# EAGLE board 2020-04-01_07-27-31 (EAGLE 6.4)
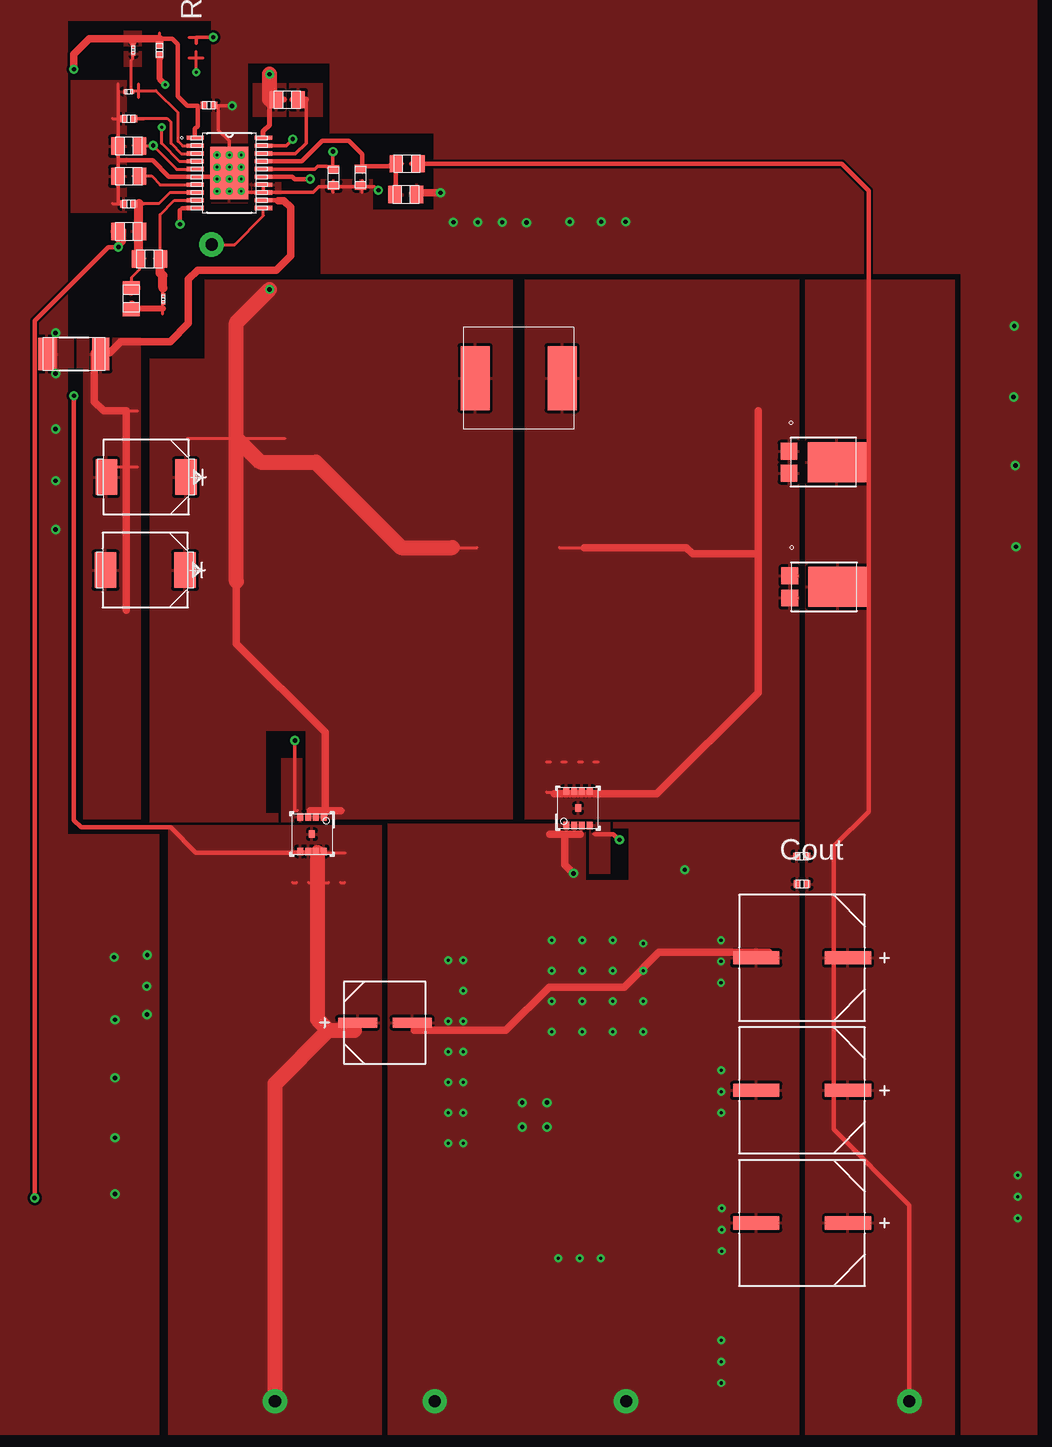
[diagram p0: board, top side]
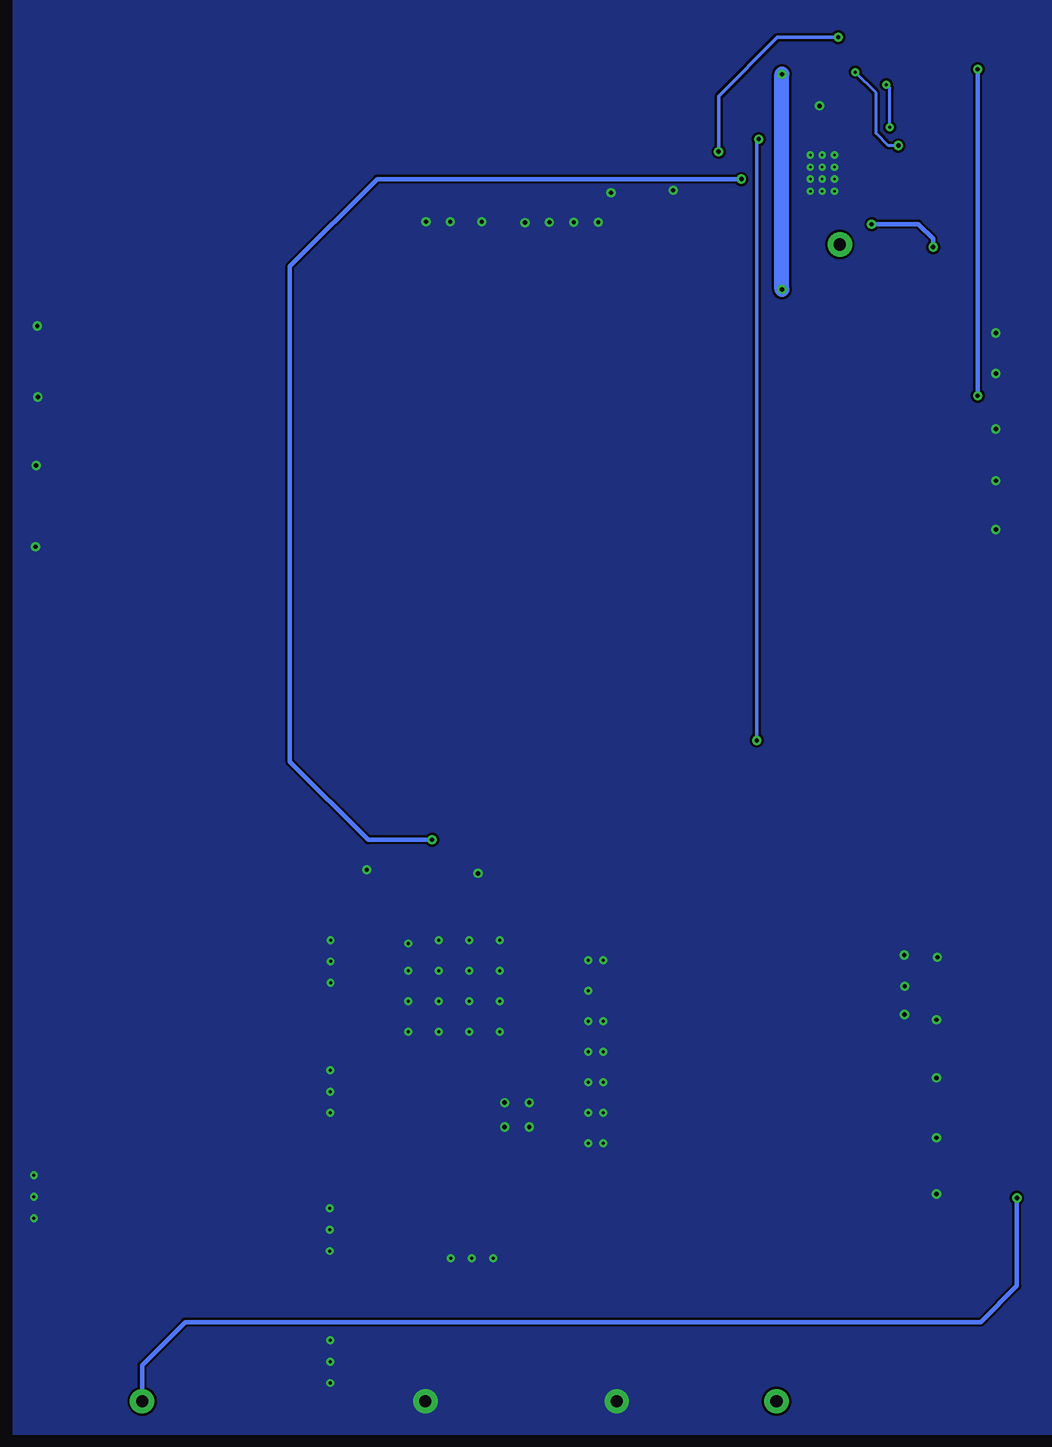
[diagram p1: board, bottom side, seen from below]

No outline drawn. Coordinates in mm, seen from the top.
Copper layers ((1*2)+(15*16)): TOP / INTERNAL1 / layer 15 / BOTTOM

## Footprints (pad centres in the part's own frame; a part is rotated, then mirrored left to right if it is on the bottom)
0805 = smd 1.118 x 1.448: 1 -0.902,0; 2 0.902,0
CAPSMT_62_C10 = smd 3.251 x 0.813: 1 -2.273,0; 2 2.273,0
0402 = smd 0.559 x 0.61: 1 -0.419,0; 2 0.419,0
CAPSMT_62_F12 = smd 3.861 x 1.092: 1 -3.823,0; 2 3.823,0
0603 = smd 0.66 x 0.965: 1 -0.699,0; 2 0.699,0
SMC = smd 1.803 x 2.972: 1 -3.315,0; 2 3.315,0
PowerDI5 = smd 1.397 x 1.397: 1 -0.92,-2.857; 3 0.92,-2.857 | smd 3.353 x 4.851: 2 0,1.13
TP-1502 = drill 0.813 round: 1 0,0
WE-LHMI_8040 = smd 2.42 x 5.33: 1 -3.62,0; 2 3.62,0
DQG0008A = smd 0.63 x 0.5: 1 -1.435,0.975; 2 -1.435,0.325; 3 -1.435,-0.325; 4 -1.435,-0.975; 5 1.435,-0.975; 6 1.435,-0.325; 7 1.435,0.325; 8 1.435,0.975; 9 0,0
0201 = smd 0.356 x 0.33: 1 -0.292,0; 2 0.292,0
2512 = smd 1.422 x 2.718: 1 -2.248,0; 2 2.248,0
MXA20A = smd 1.422 x 0.356: 1 -2.845,2.925; 2 -2.845,2.275; 3 -2.845,1.625; 4 -2.845,0.975; 5 -2.845,0.325; 6 -2.845,-0.325; 7 -2.845,-0.975; 8 -2.845,-1.625; 9 -2.845,-2.275; 10 -2.845,-2.925; 11 2.845,-2.925; 12 2.845,-2.275; 13 2.845,-1.625; 14 2.845,-0.975; 15 2.845,-0.325; 16 2.845,0.325; 17 2.845,0.975; 18 2.845,1.625; 19 2.845,2.275; 20 2.845,2.925 | smd 3.15 x 4.343: 21 0,0

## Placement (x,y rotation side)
Cboot  [0805]  51.31,137.41 0 top
Ccomp  [0805]  39.83,124.16 180 top
Ccomp2  [0805]  38.3,120.85 90 top
Cin  [CAPSMT_62_C10]  59.44,60.5 0 top
Cinx  [0402]  44.78,136.96 0 top
Cout_1  [CAPSMT_62_F12]  94.21,65.91 180 top
Cout_2  [CAPSMT_62_F12]  94.21,54.86 180 top
Cout_3  [CAPSMT_62_F12]  94.21,43.81 180 top
Coutx  [0402]  94.21,72.06 180 top
Coutx2  [0402]  94.18,74.37 180 top
Cramp  [0805]  38.1,133.55 180 top
Css  [0805]  38.1,131.04 180 top
Cvcc  [0603]  55.17,130.94 270 top
Cvccx  [0603]  57.43,130.96 90 top
D1  [SMC]  39.47,98.22 180 top
D2  [PowerDI5]  96.04,96.82 270 top
D3  [SMC]  39.55,105.97 180 top
D4  [PowerDI5]  95.99,107.21 270 top
GND  [TP-1502]  63.58,28.91 180 top
GND1  [TP-1502]  79.53,28.91 180 top
L1  [WE-LHMI_8040]  70.59,114.22 180 top
M1  [DQG0008A]  53.37,76.23 270 top
M2  [DQG0008A]  75.54,78.38 90 top
Rcomp  [0201]  40.97,120.8 270 top
Renable  [0402]  40.67,141.55 270 top
Rfbb  [0402]  38.1,128.73 180 top
Rfbt  [0805]  38.1,126.44 0 top
RHIGH  [0805]  61.29,132.08 0 top
RLOW  [0805]  61.19,129.51 180 top
Rsense  [2512]  33.53,116.23 180 top
Rt  [0402]  38.1,135.84 180 top
Ruv1  [0201]  38.48,141.55 270 top
Ruv2  [0201]  38.1,138.1 180 top
Sync  [TP-1502]  44.96,125.35 180 top
U1  [MXA20A]  46.48,131.32 0 top
VIN  [TP-1502]  50.24,28.91 180 top
VOUT  [TP-1502]  103.12,28.91 180 top

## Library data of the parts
Cboot = ultra-librarian; RefDes: Cboot; Type: 08053C104JAZ2A
Ccomp = ultra-librarian; RefDes: Ccomp; Type: CL21C222JBFNNNE
Ccomp2 = ultra-librarian; RefDes: Ccomp2; Type: 08053C104JAZ2A
Cin = ultra-librarian; RefDes: Cin; Type: 16SVPG270M
Cinx = ultra-librarian; RefDes: Cinx; Type: GRM155R71C104KA88D
Cout_1-Cout_3 Coutx Coutx2 = ultra-librarian
Cramp = ultra-librarian; RefDes: Cramp; Type: CL21C471KBANNNC
Css = ultra-librarian; RefDes: Css; Type: CGA4J2C0G1H223J125AA
Cvcc = ultra-librarian; RefDes: Cvcc; Type: C0603C105Z8VACTU
Cvccx = ultra-librarian; RefDes: Cvccx; Type: C0603C105Z8VACTU
D1 = ultra-librarian; RefDes: D1; Type: B540C-13-F
D2 = ultra-librarian; RefDes: D2; Type: PDS760-13
D3 = ultra-librarian; RefDes: D3; Type: B540C-13-F
D4 = ultra-librarian; RefDes: D4; Type: PDS760-13
GND = ultra-librarian; RefDes: GND; Type: TP-1502
GND1 = ultra-librarian; RefDes: GND1; Type: TP-1502
L1 = ultra-librarian; RefDes: L1; Type: 74437358082
M1 = ultra-librarian; RefDes: M1; Type: CSD16340Q3
M2 = ultra-librarian; RefDes: M2; Type: CSD16340Q3
Rcomp = ultra-librarian; RefDes: Rcomp; Type: RC0201FR-0712K1L
Renable = ultra-librarian; RefDes: Renable; Type: CRCW04021M00FKED
Rfbb = ultra-librarian; RefDes: Rfbb; Type: CRCW04021K00FKED
Rfbt = ultra-librarian; RefDes: Rfbt; Type: RT0805BRD073K05L
RHIGH = ultra-librarian; RefDes: RHIGH; Type: 08051A100CAT2A
RLOW = ultra-librarian; RefDes: RLOW; Type: 08051A100CAT2A
Rsense = ultra-librarian; RefDes: Rsense; Type: PMR100HZPFU10L0
Rt = ultra-librarian; RefDes: Rt; Type: CRCW040261K9FKED
Ruv1 = ultra-librarian; RefDes: Ruv1; Type: RC0201FR-0712K1L
Ruv2 = ultra-librarian; RefDes: Ruv2; Type: RC0201FR-0712K1L
Sync = ultra-librarian; RefDes: Sync; Type: TP-1502
U1 = ultra-librarian; RefDes: U1; Type: LM25118MH/NOPB
VIN = ultra-librarian; RefDes: VIN; Type: TP-1502
VOUT = ultra-librarian; RefDes: VOUT; Type: TP-1502

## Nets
0: Cin.2 Cinx.2 Cout_1.2 Cout_2.2 Cout_3.2 Coutx2.2 Coutx.2 Cramp.2 Css.2 Cvcc.2 Cvccx.1 GND1.1 GND.1 M2.1 M2.2 M2.3 Rfbb.2 RLOW.1 Rsense.2 Rt.2 Ruv2.2 U1.6 U1.13 U1.14 U1.21
1: Ruv1.2 Ruv2.1 U1.2
2: Rt.1 U1.3
3: Renable.2 U1.4
4: Cramp.1 U1.5
5: Css.1 U1.7
6: Cout_1.1 Cout_2.1 Cout_3.1 Coutx2.1 Coutx.1 Cvccx.2 D2.2 D4.2 Rfbt.1 RHIGH.1 RHIGH.2 RLOW.2 U1.10 U1.17 VOUT.1
7: Ccomp2.2 Ccomp.2 Rfbb.1 Rfbt.2 U1.8
8: Ccomp.1 Rcomp.1 U1.9
9: Cin.1 Cinx.1 M1.5 M1.6 M1.7 M1.8 M1.9 Renable.1 Ruv1.1 U1.1 VIN.1
10: Cboot.1 D1.1 D3.1 L1.2 M1.1 M1.2 M1.3 U1.20
11: D1.2 D3.2 Rsense.1 U1.12
12: M2.4 U1.15
13: Ccomp2.1 Rcomp.2
14: Cvcc.1 U1.16
15: M1.4 U1.19
16: Cboot.2 U1.18
17: D2.1 D2.3 D4.1 D4.3 L1.1 M2.5 M2.6 M2.7 M2.8 M2.9
19: Sync.1 U1.11

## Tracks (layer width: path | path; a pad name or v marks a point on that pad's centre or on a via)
0  (via drill 0.2 pad 0.48, 0.25 pad 0.61, 0.36 pad 0.71, 1.02 pad 2.03)
  TOP 0.254: 55.1,129.69 55.1,130.63 | 57.54,129.69 57.54,130.63 | 37.22,137.59 37.22,138.74 | 36.75,131.05 37.69,131.05 | 36.75,133.59 37.69,133.59 | 75.56,76.24 75.84,76.24 | 74.3,76.24 74.57,76.24 | 73.03,76.24 73.3,76.24 | 36.75,128.76 37.69,128.76 | 46.46,129.39 46.46,133.22 | 36.75,135.85 37.69,135.85
  TOP 0.305: 37.69,128.78 37.24,128.78 37.24,130.94 | 37.24,131.06 37.24,133.6 37.24,135.87 | 45.29,130.99 v45.47,130.81 | U1.13 49.33,130.33 | U1.13 47.6,129.69 v47.47,129.79 | v46.48,132.82 46.48,133.99 45.57,134.87 45.57,136.91 v46.71,136.91 | 57.56,130.18 55.12,130.18 53.95,130.18 53.47,129.69 U1.13 | 37.24,135.87 | 37.24,135.87 37.24,138.18 | v58.9,129.87 58.57,130.18 57.56,130.18 | 32,116.33 v32,117.98 | 32,116.33 | v32,114.61 32,116.33 | 57.56,130.18 57.56,130.66
  TOP 0.356: 37.39,132.36 40.08,132.36 41.43,130.99 43.61,130.99 45.29,130.99
  TOP 0.635: 91.44,66.37 82.27,66.37 79.38,63.48 73.13,63.48 69.52,59.87 61.9,59.87 | v64.08,129.67 62.08,129.67 61.77,129.67 | 73.18,76.22 74.45,76.22 | 74.45,76.22 75.72,76.22 | 74.45,76.22 74.45,73.66 v75.16,72.95
  other vias: 46.48,131.8 47.47,131.8 46.48,130.81 47.47,130.81 46.48,129.79 45.47,129.79 45.47,131.8 45.47,132.82 47.47,132.82 111.89,118.57 111.84,112.65 65.99,65.71 65.99,63.17 65.99,60.63 65.99,58.09 64.72,50.47 65.99,55.55 65.99,53.01 65.99,50.47 64.72,65.71 64.72,60.63 64.72,58.09 64.72,55.55 64.72,53.01 39.65,66.14 36.96,60.76 36.96,50.93 36.96,55.91 36.88,65.96 77.47,127.25 79.5,127.25 112.04,100.18 111.99,106.93 39.62,61.19 39.6,63.55 32,101.6 32,105.66 32,109.98 74.85,127.25 36.96,46.23 70.89,53.85 70.89,51.82 72.95,53.85 72.95,51.82 84.43,73.25 71.25,127.18 67.18,127.2 65.15,127.2 69.22,127.2 87.45,63.83 87.45,67.39 87.45,65.61 87.48,52.98 87.48,56.54 87.48,54.76 87.48,30.48 87.48,34.04 87.48,32.26 87.5,41.48 87.5,45.03 87.5,43.26 73.36,59.74 73.36,62.28 73.36,64.82 75.9,59.74 75.9,62.28 75.9,64.82 78.44,64.82 78.44,62.28 78.44,59.74 80.98,59.74 80.98,62.28 80.98,64.82 78.44,67.36 75.9,67.36 73.36,67.36 80.98,67.11 112.17,46 112.17,47.78 112.17,44.22 73.89,40.87 77.44,40.87 75.67,40.87 63.6,28.96 79.55,28.96
  pour TOP (rank 6): 42.93,130.81 42.93,131.14 44.09,131.14 44.09,130.81
  pour TOP (rank 6): 48.62,129.51 48.62,129.84 49.81,129.84 49.81,129.51
  pour TOP (rank 6): 61.42,128.91 61.42,130.4 62.71,130.4 62.71,128.91
  pour TOP: 63.5,134.62 54.86,134.62 54.86,140.46 48.01,140.46 48.01,130.56 50.8,130.56 50.8,129.54 48.01,129.54 48.01,128.78 44.96,128.78 44.96,144.02 33.02,144.02 33.02,117.6 33.53,117.6 33.53,115.06 33.02,115.06 33.02,76.2 40.64,76.2 40.64,26.16 26.16,26.16 26.16,154.18 113.79,154.18 113.79,26.16 107.44,26.16 107.44,122.94 54.1,122.94 54.1,130.81 58.42,130.81 58.42,128.27 63.5,128.27
  pour TOP: 59.69,77.09 76.2,77.09 76.2,72.39 79.76,72.39 79.76,76.71 78.49,76.71 78.49,77.22 93.98,77.22 93.98,26.16 59.69,26.16
  pour TOP: 37.92,139.04 37.92,127.99 33.27,127.99 33.27,136.4 33.27,136.93 33.27,139.04
  pour BOTTOM: 113.92,154.43 113.92,26.16 25.91,26.16 25.91,154.43
1
  TOP 0.254: 38.43,141.35 38.43,140.82 38.3,140.69 38.3,138.33 38.46,138.18 38.94,138.18 40.36,138.18 42.22,136.32 42.22,133.96 42.6,133.58 43.61,133.58 | 38.92,137.59 38.92,138.74
  pour TOP: 42.93,133.4 42.93,133.73 44.09,133.73 44.09,133.4
  pour TOP (rank 5): 37.67,140.16 37.67,141.45 39.17,141.45 39.17,140.16
2
  TOP 0.254: 43.61,132.92 42.47,132.92 41.63,133.78 41.63,135.53 41.3,135.87 38.94,135.87 38.35,135.87 | 38.46,135.85 39.4,135.85
  pour TOP (rank 2): 42.93,132.77 42.93,133.1 44.09,133.1 44.09,132.77
3  (via drill 0.25 pad 0.61)
  TOP 0.254: v40.84,135.13 40.84,133.78 42.32,132.28 43.61,132.28 | 40.68,140.34 40.68,141.28
  TOP 0.508: 40.69,141.25 40.69,140.82 40.69,139.14 v41.15,138.68
  BOTTOM 0.254: v41.15,138.68 40.84,138.38 v40.84,135.13
  pour TOP (rank 2): 42.93,132.11 42.93,132.44 44.09,132.44 44.09,132.11
4  (via drill 0.25 pad 0.61, 0.36 pad 0.71)
  TOP 0.254: 43.61,131.62 42.09,131.62 v40.13,133.6 38.94,133.6 38.61,133.6 | v43.71,139.72 43.71,140.92 43.71,141.45 | 38.46,133.59 39.4,133.59 | 43.13,140.91 44.27,140.91
  BOTTOM 0.254: v43.71,139.72 41.99,138 41.99,134.62 40.97,133.6 v40.13,133.6
  pour TOP (rank 2): 42.93,131.44 42.93,131.78 44.09,131.78 44.09,131.44
5
  TOP 0.254: 43.61,130.33 40.72,130.33 40.01,131.06 38.94,131.06 38.56,131.06 | 38.46,131.05 39.4,131.05
  pour TOP (rank 2): 42.93,130.15 42.93,130.48 44.09,130.48 44.09,130.15
6  (via drill 0.36 pad 0.71, 1.02 pad 2.03)
  TOP 0.254: 57.54,131.39 57.54,132.33 | 61.57,132.07 62.51,132.07 | 59.87,132.07 60.81,132.07
  TOP 0.356: 37.69,126.59 37.69,125.58 v37.24,125.15 | v37.24,125.15 36.4,125.15 30.25,119 v30.25,45.9 | v37.24,125.15 37.24,126.47 | 60.38,129.16 60.38,129.67 60.35,129.69 60.35,132.08 | 60.35,132.08 60.17,131.88 57.56,131.88 | 99.75,97.28 99.75,78.11 96.85,75.21 96.85,51.61 103.15,45.31 v103.15,28.96 | 99.75,97.28 | 99.75,97.28 99.75,109.22 99.75,129.84 97.54,132.08 62.05,132.08 61.62,132.08 | 57.56,131.88 57.56,132.89 56.44,134.01 54.23,134.01 52.5,132.28 U1.17 | v42.37,127.05 42.37,128.19 42.55,128.37 43.61,128.37 | 57.56,131.42 57.56,131.88 | 60.35,132.08 60.83,132.08
  BOTTOM 0.356: v42.37,127.05 38.46,127.05 37.24,125.83 v37.24,125.15 | v30.25,45.9 30.25,38.58 33.27,35.56 99.57,35.56 103.15,31.98 v103.15,28.96
  pour TOP: 36.58,125.7 36.58,127.2 37.87,127.2 37.87,125.7
  pour TOP (rank 3): 42.93,128.19 42.93,128.52 44.09,128.52 44.09,128.19
  pour TOP (rank 3): 48.62,132.11 48.62,132.44 49.81,132.44 49.81,132.11
  pour TOP (rank 4): 59.72,128.91 59.72,130.4 61.01,130.4 61.01,128.91
  pour TOP (rank 5): 94.49,122.43 106.93,122.43 106.93,26.16 94.49,26.16
7
  TOP 0.254: 38.94,128.78 | 38.94,128.78 38.91,128.75 38.41,128.75 | 43.61,129.69 41.55,129.69 40.64,128.78 38.94,128.78 | 39.01,123.29 38.35,122.63 38.35,121.74 38.35,121.23 | 39.01,123.29 | 39.01,123.29 39.01,124.21 | 38.53,124.19 39.47,124.19 | 38.46,128.76 39.4,128.76
  TOP 0.762: 38.94,128.78 38.94,126.47 38.94,124.28 39.01,124.21
  pour TOP: 38.28,125.7 38.28,127.2 39.57,127.2 39.57,125.7
  pour TOP: 37.59,121.08 37.59,122.38 39.09,122.38 39.09,121.08
  pour TOP (rank 2): 42.93,129.51 42.93,129.84 44.09,129.84 44.09,129.51
8
  TOP 0.254: 43.61,129.03 41.91,129.03 40.72,127.84 40.72,124.21 | 40.93,121.26 40.93,122.2 | 40.23,124.19 41.17,124.19
  TOP 0.762: 40.95,121.74 40.95,122.76 40.72,122.99 40.72,124.21
  pour TOP (rank 2): 42.93,128.85 42.93,129.18 44.09,129.18 44.09,128.85
9  (via drill 0.36 pad 0.71, 1.02 pad 2.03)
  TOP 0.254: 55.75,72.17 56.08,72.17 | 54.43,72.17 54.76,72.17 | 53.09,72.17 53.42,72.17 | 51.77,72.17 52.09,72.17 | 51.77,74.66 56.11,74.66 | 40.68,142.04 40.68,142.98
  TOP 0.356: 40.69,142.52 41.71,142.52 42.19,142.04 42.19,137.69 42.98,136.91 43.87,136.91 43.87,135.23 43.61,135 43.61,134.24 | 53.85,74.68 43.69,74.68 41.6,76.78 34.14,76.78 33.53,77.39 v33.53,112.75
  TOP 0.635: v33.53,139.95 33.53,141.22 34.82,142.52 38.43,142.52 | 38.43,142.19 38.43,142.52 | 40.69,142.19 40.69,142.52 38.43,142.52 | 40.69,142.19
  TOP 1.27: 53.85,74.68 53.85,60.76 54.74,59.87 | 54.74,59.87 56.9,59.87 | 54.74,59.87 50.29,55.42 v50.29,28.96
  BOTTOM 0.356: v33.53,112.75 v33.53,139.95
  pour TOP: 42.93,134.06 42.93,134.39 44.09,134.39 44.09,134.06
  pour TOP (rank 5): 37.67,141.86 37.67,143.15 39.17,143.15 39.17,141.86
  pour TOP (rank 6): 59.18,26.16 59.18,76.96 41.4,76.96 41.4,26.16
10  (via drill 0.36 pad 0.71)
  TOP 0.254: 53.16,78.17 53.44,78.17 | 54.43,78.17 54.71,78.17 | 55.7,78.17 55.98,78.17 | 62.99,100.09 67.13,100.09 | 43,109.21 51.13,109.21
  TOP 0.406: 49.84,137.44 49.84,135.33 49.33,134.85 U1.20
  TOP 0.508: 49.84,137.44 51.03,137.44 | 51.03,137.44
  TOP 0.635: 54.48,78.18 55.75,78.18 | 54.48,78.18 54.48,84.71 47.07,92.1 47.07,97.28 | 54.48,78 54.48,78.18 | 53.21,78.18 54.3,78.18
  TOP 1.27: 49.84,137.44 v49.84,139.55 | 47.07,97.28 47.07,109.22 | 47.07,109.22 49.07,107.21 53.7,107.21 60.81,100.1 65.08,100.1 | 47.07,109.22 47.07,118.85 v49.84,121.61
  BOTTOM 1.27: v49.84,121.61 v49.84,139.55
  pour TOP (rank 3): 48.62,134.06 48.62,134.39 49.81,134.39 49.81,134.06
  pour TOP (rank 4): 48.44,136.02 48.44,138.81 51.23,138.81 51.23,136.02
  pour TOP (rank 5): 70.1,77.47 70.1,122.43 44.45,122.43 44.45,115.82 39.85,115.82 39.85,77.22 50.55,77.22 50.55,77.98 49.53,77.98 49.53,84.84 52.83,84.84 52.83,77.47
11
  TOP 0.254: 36.91,111.48 38.81,111.48 | 36.91,106.83 38.81,106.83
  TOP 0.381: U1.12 50.55,129.03
  TOP 0.635: 50.55,129.01 51.03,129.01 51.59,128.47 51.59,124.41 50.39,123.22 43.84,123.22 43.08,122.45 43.08,118.8 41.55,117.27 37.44,117.27 36.5,116.33 35.23,116.33 35.23,112.27 36.02,111.48 37.87,111.48 37.87,106.83 37.87,99.54 37.87,94.89
  pour TOP (rank 4): 48.62,128.85 48.62,129.18 49.81,129.18 49.81,128.85
  pour TOP (rank 5): 39.12,117.6 39.12,77.47 34.29,77.47 34.29,115.06 33.78,115.06 33.78,117.6
12  (via drill 0.36 pad 0.71)
  TOP 0.254: 76.83,76.24 77.11,76.24
  TOP 0.356: v78.99,75.74 78.49,76.22 76.99,76.22 | v53.21,130.81 51.94,130.81 51.74,130.99 U1.15
  BOTTOM 0.356: v78.99,75.74 84.33,75.74 90.83,82.25 90.83,123.55 83.57,130.81 v53.21,130.81
  pour TOP (rank 4): 48.62,130.81 48.62,131.14 49.81,131.14 49.81,130.81
  pour TOP (rank 5): 76.45,77.22 78.23,77.22 78.23,72.9 76.45,72.9
13
  TOP 0.254: 40.93,119.56 40.93,120.5
  TOP 0.508: 40.95,120.04 38.35,120.04 38.35,120.45 | 38.35,120.45
  pour TOP: 37.59,119.38 37.59,120.68 39.09,120.68 39.09,119.38
14  (via drill 0.36 pad 0.71)
  TOP 0.254: 55.1,131.39 55.1,132.33 | 43.13,142.61 44.27,142.61
  TOP 0.305: v45.14,142.62 | v55.12,133.1 55.12,131.88 55.12,131.39 | 49.33,131.62 53.59,131.62 53.85,131.88 54.61,131.88 55.12,131.39 | v45.14,142.62 43.71,142.62 43.71,142.14 | 55.12,131.39
  BOTTOM 0.305: v45.14,142.62 50.22,142.62 55.12,137.72 v55.12,133.1
  pour TOP (rank 3): 48.62,131.44 48.62,131.78 49.81,131.78 49.81,131.44
15  (via drill 0.36 pad 0.71)
  TOP 0.254: 51.89,78.17 52.17,78.17
  TOP 0.305: v51.94,84.02 | 51.94,78.18 v51.94,84.02 | v51.77,134.14 51.21,133.58 U1.19
  BOTTOM 0.305: v51.77,134.14 51.94,133.96 v51.94,84.02
  pour TOP (rank 3): 48.62,133.4 48.62,133.73 49.81,133.73 49.81,133.4
  pour TOP (rank 6): 50.8,82.55 52.58,82.55 52.58,77.22 50.8,77.22
16
  TOP 0.305: 49.33,132.92 51.99,132.92 52.88,133.81 52.88,137.44
  TOP 0.508: 51.74,137.44 52.88,137.44 | 51.74,137.44
  pour TOP (rank 3): 48.62,132.77 48.62,133.1 49.81,133.1 49.81,132.77
  pour TOP (rank 4): 51.49,136.02 51.49,138.81 54.28,138.81 54.28,136.02
17
  TOP 0.254: 72.9,82.23 73.23,82.23 | 74.22,82.23 74.55,82.23 | 75.56,82.23 75.89,82.23 | 76.89,82.23 77.22,82.23 | 72.9,79.72 77.24,79.72 | 73.99,100.09 78.13,100.09
  TOP 0.635: 90.55,111.48 90.55,106.83 90.55,99.19 | 76.07,100.1 84.56,100.1 85.09,99.57 90.55,99.57 90.55,99.54 90.55,99.19 | 90.55,99.19 | 90.55,99.19 90.55,94.89 90.55,88.01 82.27,79.73 82.12,79.58 80.77,79.58 73.56,79.58
  pour TOP (rank 6): 93.95,122.43 93.95,77.47 71.12,77.47 71.12,122.43
19  (via drill 1.02 pad 2.03)
  TOP 0.254: v45.01,125.35 46.91,125.35 49.33,127.76 49.33,128.37
  pour TOP (rank 4): 48.62,128.19 48.62,128.52 49.81,128.52 49.81,128.19

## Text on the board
ASSYNOTES: Rramp | Cout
